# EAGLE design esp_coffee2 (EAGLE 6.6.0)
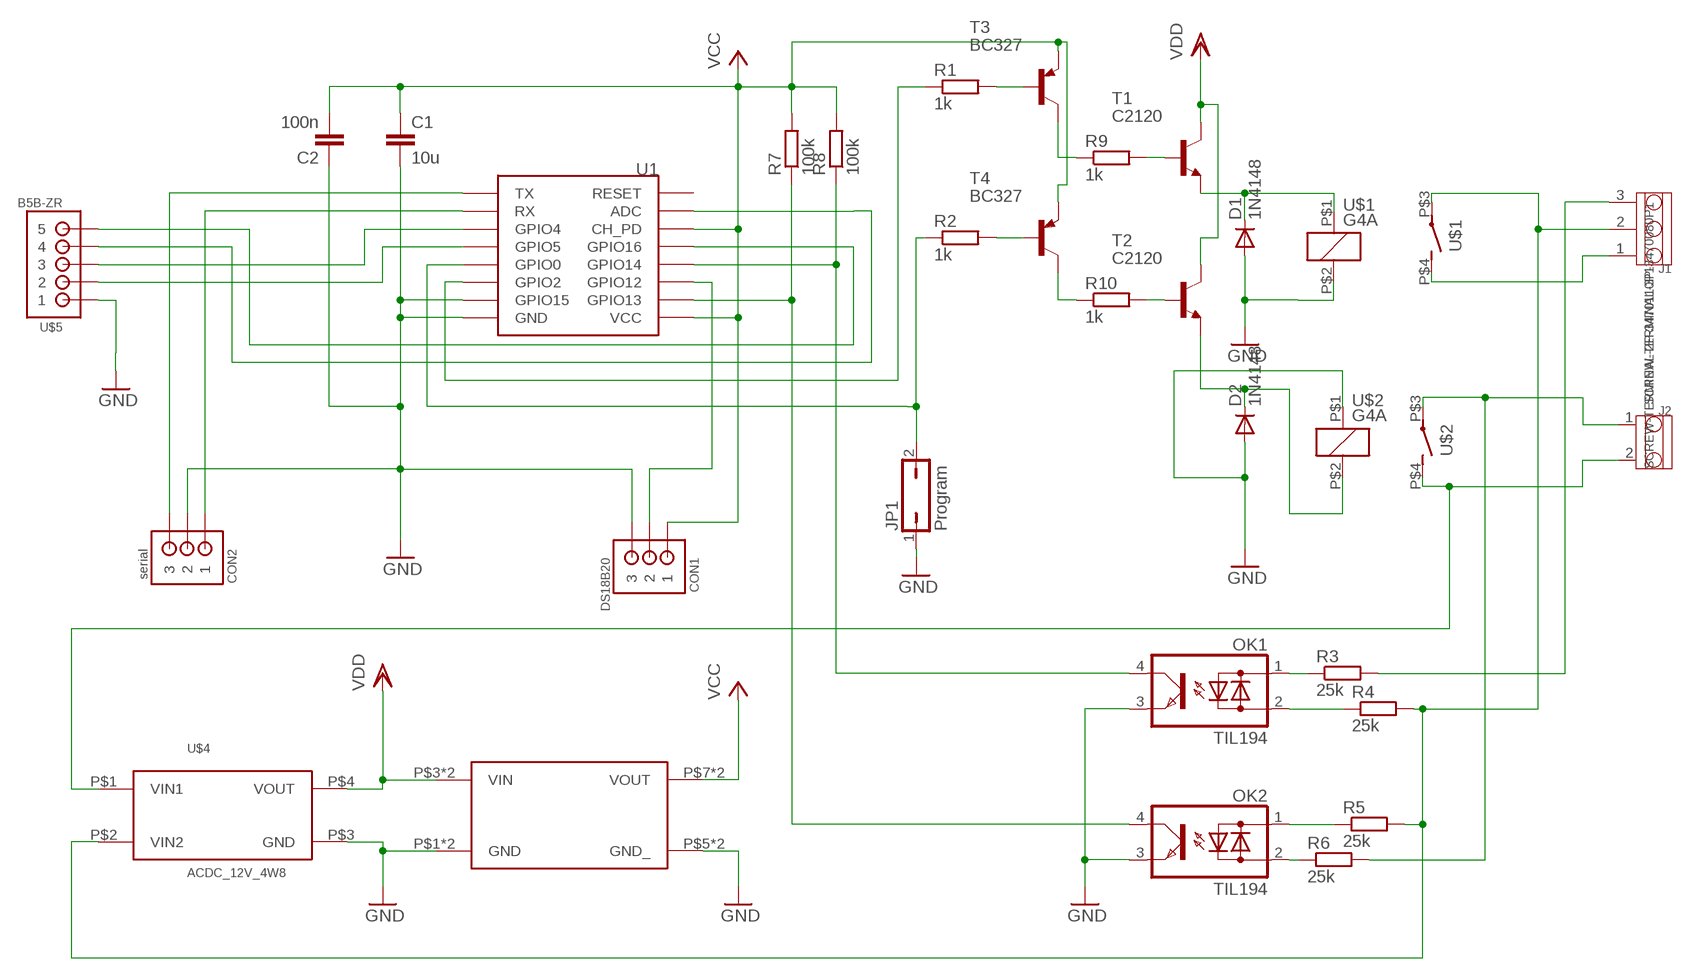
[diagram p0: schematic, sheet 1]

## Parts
C1  10u  C-EUC0603K  [C0603K]
C2  100n  C-EUC1206  [C1206]
CON1  DS18B20  B3B-ZR  [B3B-ZR]
CON2  serial  B3B-ZR  [B3B-ZR]
D1  1N4148  1N4148DO35-10  [DO35-10]
D2  1N4148  1N4148DO35-10  [DO35-10]
J1  SCREW-TERMINAL-3P-3470080P1  [3P-5.0]
J2  SCREW-TERMINAL-2P-3470110P1  [2P-5.0]
JP1  Program  JP1Q  [JP1]
OK1  TIL194  [DIL04]
OK2  TIL194  [DIL04]
R1  1k  R-EU_R0603  [R0603]
R2  1k  R-EU_R0603  [R0603]
R3  25k  R-EU_R0603  [R0603]
R4  25k  R-EU_R0603  [R0603]
R5  25k  R-EU_R0603  [R0603]
R6  25k  R-EU_R0603  [R0603]
R7  100k  R-EU_R0603  [R0603]
R8  100k  R-EU_R0603  [R0603]
R9  1k  R-EU_R0603  [R0603]
R10  1k  R-EU_R0603  [R0603]
T1  C2120  -NPN-TO92-ECB  [TO92-ECB]
T2  C2120  -NPN-TO92-ECB  [TO92-ECB]
T3  BC327  BC327-16-PNP-TO92-EBC  [TO92-EBC]
T4  BC327  BC327-16-PNP-TO92-EBC  [TO92-EBC]
U1  ESP12SMD  [ESP12-SMD]
U$1  G4A  [G4A]
U$2  G4A  [G4A]
U$3  DCDC_MP1584  [DCDC_MP1584_DOWN]
U$4  ACDC_12V_4W8  [ACDC_4W8]
U$5  B5B-ZR  [B5B-ZR]

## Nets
ADC: U1.ADC U$5.4
BLUE: J1.2 R4.2 R5.2 U$1.P$3(S:P) U$4.P$2(VIN2)
BROWN/BLACK: J2.2 U$2.P$4(S:S) U$4.P$1(VIN1)
GND: C1.2 C2.1 CON1.3 CON2.2 D1.A D2.A JP1.1 OK1.3(E) OK2.3(E) U1.GND U1.GPIO15 U$1.P$2 U$2.P$1 U$3.P$1(GND) U$3.P$2(GND) U$3.P$5(GND_) U$3.P$6(GND_) U$4.P$3(GND) U$5.1
GPIO0: JP1.2 R2.1 U1.GPIO0
GPIO2: R1.1 U1.GPIO2
GPIO4: U1.GPIO4 U$5.3
GPIO5: U1.GPIO5 U$5.2
GPIO12: CON1.2 U1.GPIO12
GPIO13: OK2.4(C) R7.1 U1.GPIO13
GPIO14: OK1.4(C) R8.1 U1.GPIO14
GPIO16: U1.GPIO16 U$5.5
GREY: J1.1 U$1.P$4(S:S)
HEAT: J1.3 R3.2
N$1: R9.2 T1.B
N$2: D1.C T1.E U$1.P$1
N$3: D2.C T2.E U$2.P$2
N$4: R10.2 T2.B
N$5: R10.1 T4.C
N$6: R9.1 T3.C
N$7: R2.2 T4.B
N$8: R1.2 T3.B
N$14: OK2.1(AC1) R5.1
N$15: OK2.2(AC2) R6.1
N$17: OK1.2(AC2) R4.1
N$18: OK1.1(AC1) R3.1
ORANGE/RED: J2.1 R6.2 U$2.P$3(S:P)
RX: CON2.1 U1.RXD0(RX)
TX: CON2.3 U1.TXD0(TX)
VCC: C1.1 C2.2 CON1.1 R7.2 R8.2 T3.E T4.E U1.CH_PD U1.VCC U$3.P$7(VOUT) U$3.P$8(VOUT)
VDD: T1.C T2.C U$3.P$3(VIN) U$3.P$4(VIN) U$4.P$4(VOUT)
Unconnected: U1.RESET

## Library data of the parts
C1 C2 = 00Eigene:C-EU: CAPACITOR, European symbol
CON1 CON2 = jst:B3B-ZR: JST-ZH Connector 3 pol, 1.5mm pitch Package: B3B-ZR Source: http://www.jst-mfg.com/product/pdf/eng/eZH.pdf
D1 D2 = diode:1N4148: DIODE
J1 = OPL:SCREW-TERMINAL-3P
J2 = OPL:SCREW-TERMINAL-2P
JP1 = jumper:JP1Q: JUMPER
OK1 OK2 = optocoupler:TIL194: TEXAS INSTRUMENTS OPTO COUPLER; OC_FARNELL: unknown; OC_NEWARK: unknown
R1-R10 = 00Eigene:R-EU_: RESISTOR, European symbol
T1 T2 = transistor:*-NPN-: NPN Transistror BF959 corrected 2008.03.06
T3 T4 = transistor:*-PNP-: PNP Transistror
U1 = ESP8266_modules:ESP12: ESP8266 Wifi module 12
U$1 U$2 = 00Eigene:G4A: Compact Single-pole Relay for Switching 20 A Source: http://www.omron.com/ecb/products/pry/121/g5sb.html; OC_FARNELL: unknown; OC_NEWARK: unknown
U$3 = 00Eigene:DCDC_MP1584
U$4 = 00Eigene:ACDC_12V_4W8: AC DC 12V 400mA
U$5 = jst:B5B-ZR: JST-ZH Connector 5 pol, 1.5mm pitch Package: B5B-ZR Source: http://www.jst-mfg.com/product/pdf/eng/eZH.pdf

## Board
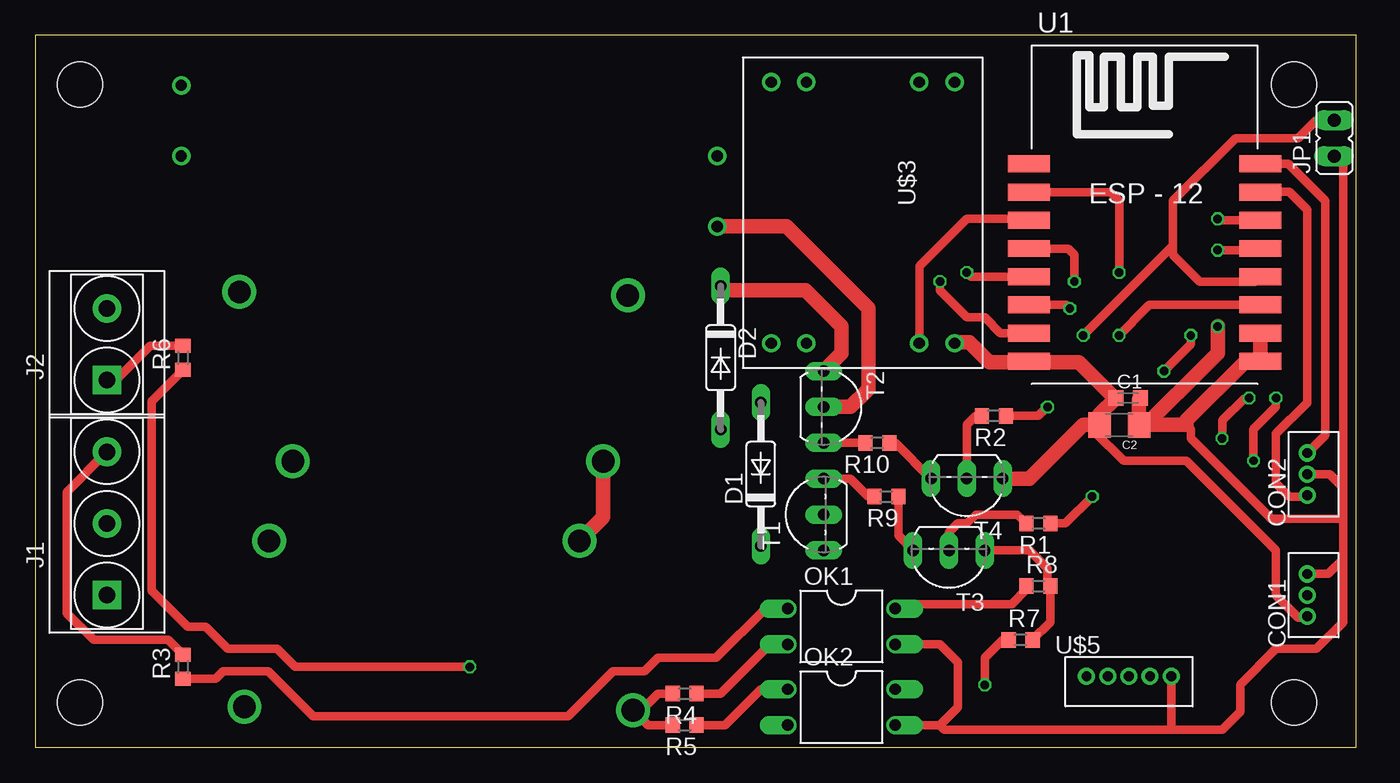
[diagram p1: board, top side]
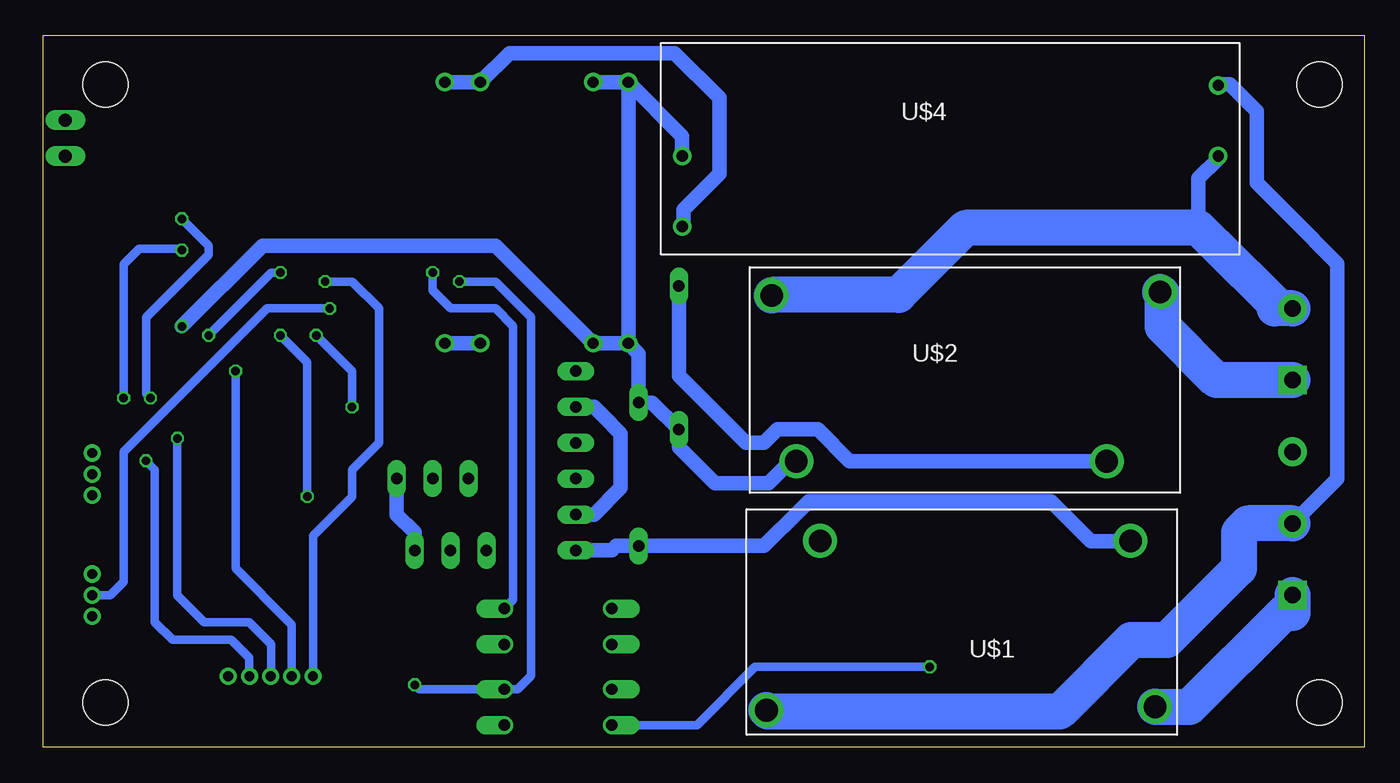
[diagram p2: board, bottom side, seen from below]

Size 93.64 x 50.47 mm. Coordinates in mm from the lower left corner, seen from the top.
Outline: 0,0 93.64,0 93.64,50.47 0,50.47 0,0
Copper layers (1*16): Top 0.035mm / dielectric 1.5mm / Bottom 0.035mm
Design rules "SeeedStudio_2layer_DRU_no_angle_20140221": minimum track width 6mil, minimum drill 12mil, track to track 6mil, track to pad 6mil, pad to pad 6mil, via to via 6mil, smd to smd 0mil, copper to edge 10mil, drill to drill 10mil, minimum pad ring 10mil, minimum via ring 6mil, stop-mask expansion 2mil, vias tented up to drill 100mil, thermal gap 10mil
Holes 3.2 mm at 3.17,46.99 89.22,46.99 89.22,3.17 3.17,3.17

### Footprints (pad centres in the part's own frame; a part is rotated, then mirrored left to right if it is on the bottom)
C0603K = smd 1.05 x 1.08: 1 -0.875,0; 2 0.875,0
C1206 = smd 1.6 x 1.8: 1 -1.4,0; 2 1.4,0
B3B-ZR = drill 0.7 pad 1.1: 1 -1.5,0; 2 0,0; 3 1.5,0
DO35-10 = drill 0.813 long: A 5.08,0; C -5.08,0
3P-5.0 = drill 1.168 pad 2.032 square: 1 -5.08,0 | drill 1.168 pad 2.032: 2 0,0; 3 5.08,0
2P-5.0 = drill 1.168 pad 2.032 square: 1 -2.54,0 | drill 1.168 pad 2.032: 2 2.54,0
JP1 = drill 0.914 long: 1 0,-1.27; 2 0,1.27
DIL04 = drill 0.813 offset: 1 -1.27,-3.81; 2 1.27,-3.81; 3 1.27,3.81; 4 -1.27,3.81
R0603 = smd 1 x 1.1: 1 -0.85,0; 2 0.85,0
TO92-ECB = drill 0.813 long: B 2.54,0; C 0,0; E -2.54,0
TO92-EBC = drill 0.813 long: B 0,-1.27; C 2.54,-1.27; E -2.54,-1.27
ESP12-SMD = smd 3 x 1.2: ADC -8.3,3.8; CH_PD -8.3,1.8; GND 8.1,-8.2; GPIO0 8.1,-2.2; GPIO2 8.1,-4.2; GPIO4 8.1,1.8; GPIO5 8.1,-0.2; GPIO12 -8.3,-4.2; GPIO13 -8.3,-6.2; GPIO14 -8.3,-2.2; GPIO15 8.1,-6.2; GPIO16 -8.3,-0.2; RESET -8.3,5.8; RXD0 8.1,3.8; TXD0 8.1,5.8; VCC -8.3,-8.2
G4A = drill 1.6: P$1 -12,-5.75; P$2 10,-5.75; P$3 13.8,6.25; P$4 -13.75,6
DCDC_MP1584_DOWN = drill 0.8: P$1 1.75,2; P$2 1.75,4.5; P$3 1.75,12.5; P$4 1.75,15; P$5 20.25,2; P$6 20.25,4.5; P$7 20.25,12.5; P$8 20.25,15
ACDC_4W8 = drill 0.8: P$1 39.5,7; P$2 39.5,12; P$3 1.5,7; P$4 1.5,2
B5B-ZR = drill 0.7: 1 7.5,-1.3; 2 6,-1.3; 3 4.5,-1.3; 4 3,-1.3; 5 1.5,-1.3

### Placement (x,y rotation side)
C1  77.47,24.77 0 top
C2  76.83,22.86 180 top
CON1  90.17,10.79 90 top
CON2  90.17,19.37 90 top
D1  51.44,19.37 90 top
D2  48.58,27.62 270 top
J1  5.08,15.88 90 top
J2  5.08,28.57 90 top
JP1  92.08,43.18 0 top
OK1  57.15,8.57 270 top
OK2  57.15,2.86 270 top
R1  71.12,15.88 180 top
R2  67.94,23.5 180 top
R3  10.48,5.71 90 top
R4  46.04,3.81 180 top
R5  46.04,1.59 180 top
R6  10.48,27.62 90 top
R7  69.85,7.62 0 top
R8  71.12,11.43 0 top
R9  60.33,17.78 180 top
R10  59.69,21.59 180 top
T1  55.88,16.51 90 top
T2  55.88,24.13 270 top
T3  64.77,12.7 180 top
T4  66.04,17.78 180 top
U1  78.74,35.56 0 top
U$1  28.57,8.89 180 bottom
U$2  28.26,26.04 0 bottom
U$3  50.16,48.9 270 top
U$4  49.85,34.92 0 bottom
U$5  73.03,6.35 0 top

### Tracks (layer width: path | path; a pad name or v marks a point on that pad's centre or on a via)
ADC  (via drill 0.6)
  Top 0.61: U1.ADC 76.21,39.36 76.83,38.73 v76.83,33.66 | v81.92,29.21 81.92,28.57 v80.01,26.67
  Bottom 0.61: v76.83,33.66 77.47,33.66 v81.92,29.21 | v80.01,26.67 80.01,12.7 76.2,8.89 76.03,8.71 U$5.4
BLUE
  Top 0.61: R4.2 44.13,3.81 42.96,2.64 U$1.P$3 43.43,1.59 R5.2
  Bottom 1.016: J1.2 1.91,19.05 1.91,34.29 5.14,37.53 7.62,40.01 7.62,44.83 7.62,45.09 9.53,46.99 10.28,46.99 U$4.P$2
  Bottom 2.54: U$1.P$3 42.27,2.54 21.59,2.54 16.51,7.62 13.97,7.62 8.89,12.7 8.89,13.97 8.89,15.24 8.26,15.88 J1.2
BROWN/BLACK
  Bottom 1.016: 12.06,36.83 11.75,37.15 11.75,40.32 10.35,41.72 U$4.P$1
  Bottom 2.54: J2.2 6.35,31.11 6.35,31.43 10.48,35.56 11.75,36.83 12.06,36.83 28.26,36.83 33.02,32.07 41.98,32.07 U$2.P$4
GND  (via drill 0.6)
  Top 0.61: CON2.2 91.76,19.37 92.71,18.41 | 92.71,18.41 92.71,16.51 | 92.71,16.51 92.71,15.24 92.71,13.34 | CON1.3 91.67,12.29 92.71,13.34 | OK2.3 64.14,1.59 | 64.14,1.59 65.41,2.86 65.41,6.03 64.14,7.3 OK1.3 | 92.71,13.34 92.71,9.21 92.71,8.89 90.81,6.99 87.95,6.99 85.41,4.45 85.41,2.54 84.14,1.27 80.64,1.27 | 92.71,16.51 92.39,16.19 87.63,16.19 83.82,20 81.92,21.91 81.92,22.54 81.6,22.86 | 80.64,1.27 64.45,1.27 64.14,1.59 | U$5.1 80.53,1.39 80.64,1.27 | JP1.1 92.71,41.27 92.71,18.41
  Top 1.016: C2.1 78.23,24.66 C1.2 | C2.1 78.74,22.86 80.01,24.13 81.92,26.04 | U1.GPIO15 U1.GND 86.78,27.3 85.72,27.3 81.6,23.18 81.6,22.86 C2.1 | 81.92,26.04 82.23,26.35 | U$2.P$1 40.26,16.32 U$1.P$2 | v83.82,29.84 83.82,27.94 81.92,26.04
  Bottom 1.016: U$3.P$5 U$3.P$1 | U$3.P$1 U$3.P$2 | U$3.P$5 U$3.P$6 61.58,35.56 67.63,35.56 75.56,35.56 76.2,35.56 78.11,35.56 v83.82,29.84 | U$3.P$5 51.44,27.91 D1.A 50.48,24.45 D2.A 48.58,21.27 46.04,18.73 42.23,18.73 40.67,20.29 U$2.P$1 | U$4.P$3 48.35,43.33 U$3.P$1
GPIO0  (via drill 0.6)
  Top 0.61: JP1.2 90.81,44.45 89.53,43.18 85.09,43.18 80.64,38.73 80.64,35.56 | 80.64,35.56 80.64,34.92 82.55,33.02 86.5,33.02 U1.GPIO0 | R2.1 71.12,23.5 v71.75,24.13 | v74.3,29.21 80.64,35.56
  Bottom 0.61: v71.75,24.13 71.75,26.67 v74.3,29.21
GPIO2  (via drill 0.6)
  Top 0.61: R1.1 73.03,15.88 v74.93,17.78 | v76.83,29.21 78.74,31.11 78.98,31.36 U1.GPIO2
  Bottom 0.61: v74.93,17.78 74.93,27.3 v76.83,29.21
GPIO4  (via drill 0.6)
  Top 0.61: v86.04,24.77 85.72,24.77 84.14,23.18 v84.14,21.91 | U1.GPIO4 83.92,37.36 v83.82,37.47
  Bottom 0.61: v84.14,21.91 84.14,10.79 82.23,8.89 79.06,8.89 77.47,7.3 77.47,5.74 77.47,5.11 U$5.3 | v83.82,37.47 81.92,35.56 81.92,34.92 86.36,30.48 86.36,25.08 v86.04,24.77
GPIO5  (via drill 0.6)
  Top 0.61: v86.36,20.32 86.36,22.54 87.95,24.13 v87.95,24.77 | v83.82,35.24 86.72,35.24 U1.GPIO5
  Bottom 0.61: v86.36,20.32 85.72,19.68 85.72,8.89 84.45,7.62 80.33,7.62 79.06,6.35 79.06,5.08 U$5.2 | v87.95,24.77 87.95,34.25 U1.GPIO5 83.94,35.36 v83.82,35.24
GPIO12  (via drill 0.6)
  Top 0.61: U1.GPIO12 73.1,31.36 v73.34,31.11
  Bottom 0.61: v73.34,31.11 77.79,31.11 84.45,24.45 87.95,20.95 87.95,11.75 88.9,10.79 CON1.2
GPIO13  (via drill 0.6)
  Top 0.61: v67.31,4.45 67.31,6.35 68.58,7.62 R7.1 | v64.14,33.02 64.14,32.38 66.04,30.48 67.31,30.48 68.43,29.36 U1.GPIO13
  Bottom 0.61: v67.31,4.45 66.99,4.13 OK2.4 60.01,4.13 59.05,5.08 59.05,30.48 61.59,33.02 v64.14,33.02
GPIO14  (via drill 0.6)
  Top 0.61: R8.1 70.27,11.21 69.22,10.16 61.28,10.16 OK1.4 | U1.GPIO14 66.33,33.36 v66.04,33.66
  Bottom 0.61: v66.04,33.66 66.04,32.38 65.41,31.75 64.77,31.11 61.59,31.11 60.33,29.84 60.33,10.48 OK1.4
GPIO16  (via drill 0.6)
  Top 0.61: v73.66,33.02 73.66,34.29 73.66,34.92 73.22,35.36 U1.GPIO16
  Bottom 0.61: U$5.5 74.53,15.01 71.75,17.78 71.75,19.68 69.85,21.59 69.85,29.84 69.85,31.11 71.75,33.02 v73.66,33.02
GREY
  Bottom 2.54: J1.1 5.08,9.53 5.71,9.53 12.38,2.86 14.79,2.86 U$1.P$4
HEAT
  Top 0.61: J1.3 2.22,18.1 2.22,9.53 4.13,7.62 9.42,7.62 R3.2
N$1
  Top 0.61: R9.2 59.05,17.78 57.78,19.05 T1.B
N$2
  Bottom 1.016: U$1.P$1 16.61,14.61 19.37,14.61 22.23,17.46 39.37,17.46 40.01,16.83 42.55,14.29 D1.C 53.02,14.29 53.34,13.97 T1.E
N$3
  Top 1.016: T2.E 57.15,27.94 57.15,29.84 56.52,30.48 54.61,32.38 48.9,32.38 D2.C
  Bottom 1.016: U$2.P$2 36.48,20.29 38.73,22.54 41.59,22.54 42.55,21.59 43.81,21.59 48.58,26.35 D2.C
N$4
  Top 0.61: R10.2 T2.B
N$5
  Top 0.61: R10.1 60.96,21.59 T4.C
N$6
  Top 0.61: R9.1 61.17,15.03 T3.C
N$7
  Top 0.61: R2.2 66.67,23.5 66.04,22.86 T4.B
N$8
  Top 0.61: T3.B 64.77,15.24 65.41,15.88 66.04,15.88 66.67,16.51 69.64,16.51 R1.2
N$14
  Top 0.61: R5.1 48.9,1.59 51.44,4.13 OK2.1
N$15  (via drill 0.6)
  Top 0.61: v30.8,5.71 18.41,5.71 17.14,6.99 13.65,6.99 13.02,7.62 12.06,8.57 10.79,8.57 8.26,11.11 8.26,21.69 8.26,24.55 R6.1
  Bottom 0.61: OK2.2 47.31,1.59 43.18,5.71 v30.8,5.71
N$17
  Top 0.61: OK1.2 52.07,7.3 50.8,6.03 48.58,3.81 R4.1
N$18
  Top 0.61: R3.1 12.8,4.87 13.34,5.4 16.51,5.4 19.68,2.22 37.78,2.22 40.96,5.4 43.18,5.4 44.13,6.35 48.26,6.35 51.75,9.84 OK1.1
ORANGE/RED
  Top 0.61: R6.2 8.15,28.47 5.71,26.04 J2.1
  Bottom 0.61: 10.48,26.04 10.48,25.93
  Bottom 2.54: J2.1 10.48,26.04 14.29,29.84 14.29,32.12 U$2.P$3
RX
  Top 0.61: CON2.1 90.08,17.78 88.9,17.78 87.95,18.73 87.95,22.23 90.17,24.45 90.17,38.1 89.53,38.73 88.9,39.37 U1.RXD0 | U1.RXD0
TX
  Top 0.61: U1.TXD0 88.81,41.36 91.44,38.73 91.44,22.14 CON2.3
VCC
  Top 0.61: C2.2 74.93,22.36 75.12,22.36 77.15,20.32 81.6,20.32 87.95,13.97 87.95,10.79 89.53,9.21 90.08,9.21 CON1.1 | 70.33,37.47 U1.CH_PD 70.33,37.47 | 70.33,37.47 66.99,37.47 66.04,37.47 62.66,34.09 U$3.P$7 | R7.2 71.97,8.89 R8.2 71.75,11.64 71.75,12.7 70.48,13.97 T3.E
  Top 0.813: 65.09,28.72 U$3.P$8
  Top 1.016: 70.39,27.3 69.85,27.3 73.98,27.3 76.52,24.77 C1.1 75.44,23.61 C2.2 74.3,22.86 70.48,19.05 T4.E | 70.39,27.3 U1.VCC 70.39,27.3 | 65.09,28.72 66.21,28.72 67.63,27.3 70.39,27.3
  Bottom 1.016: U$3.P$7 U$3.P$8 | T4.E 68.58,16.51 67.31,15.24 T3.E | T3.E 67.31,13.34 T3.E
VDD
  Top 1.016: U$4.P$4 53.24,36.92 59.05,31.11 59.05,25.4 57.78,24.13 T2.C
  Bottom 1.016: U$3.P$4 U$3.P$3 60.6,49.21 48.9,49.21 45.72,46.04 45.72,40.64 48.26,38.1 48.26,37.01 U$4.P$4 | T1.C 54.61,16.51 52.7,18.41 52.7,22.23 53.98,23.5 54.61,24.13 T2.C | T2.C 56.52,24.13 T2.C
